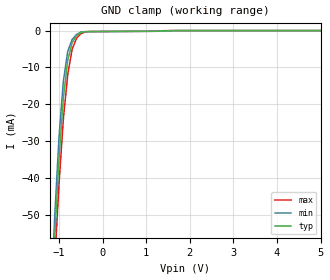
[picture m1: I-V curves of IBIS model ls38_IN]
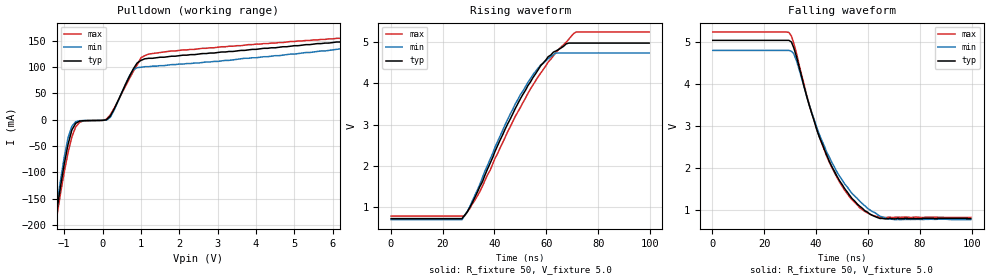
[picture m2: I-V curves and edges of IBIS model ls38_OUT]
| TEXAS INSTRUMENTS INCORPORATED
| Standard Linear and Logic Group
| IBIS Model of SN74LS38
| QUADRUPLE 2-INPUT POSITIVE-NAND BUFFERS WITH OPEN-COLLECTOR OUTPUTS
| SOP 14-pin (NS), SOIC 14-pin (D), P-DIP 14-pin (N)
[IBIS Ver]   3.2
[Comment Char] |_char
[File Name]   sn74ls38.ibs
[File Rev]   2.1 I_die
[Date]   Nov.15, 2004
[Source]   File originated at Texas Instruments, Inc.
[Notes]   The following is a sample IBIS file for the LS38.
   - FILE REV HISTORY
   - 3.2 Re-Release IBIS file on 11/16/04
   - Power clamp data deleted as there is no power-clamp diode.
|   - All test data contained in this file are derived from
|   actual measurements.
|   - File created by Nobuhisa Ohtsubo, SLL Product Engineering.
[Disclaimer] Property of Texas Instruments Incorporated.  Unauthorized
   reproduction and/or distribution is strictly prohibited.
   This product is protected under copyright law.
   Created 2000, (C) Copyright 2000, Texas Instruments Inc.,
   All Rights Reserved.
   UNLESS THERE IS A SIGNED, WRITTEN AGREEMENT TO THE
   CONTRARY, TEXAS INSTRUMENTS () IS PROVIDING THE IBIS
   MODELS  AND WITHOUT ANY WARRANTY, EXPRESSED OR
   IMPLIED.  TI assumes no liability for:
   1) the accuracy of the IBIS models provided to your
   company;
   2) the proper functioning of these IBIS Models in your
   design or for any resulting applications; or
   3) infringement of patents, copyrights or intellectual
   property rights resulting from your use of these IBIS
   models.
   TI provides IBIS Models as a service to our customers.
   You and your company shall not distribute, sell or give
   these models to anyone else without prior written
   permission from TI.
   TI reserves the right to make changes to our products or
   to discontinue any semiconductor product or service
   without notice, and advises our customers to obtain the
   latest version of relevant information to verify, before
   placing orders, that the information being relied on is
   current.
   Please be aware that your receipt and use of the IBIS
   information provided shall serve as acceptance of these
   terms and conditions.  If you do not accept these terms,
   you should return or destroy the IBIS models and any
   other accompanying information immediately.
|   Component LS38_NS
[Component]   ls38_NS
[Manufacturer]  Texas Instruments, Inc.
[Package]
|   typ   min   max
R_pkg   0.045   0.039   0.054
L_pkg   3.796nH   2.561nH   4.952nH
C_pkg   0.528pF   0.288pF   0.710pF
[Pin]   signal_name   model_name   R_pin   L_pin   C_pin
1   1A   ls38_IN   0.047   4.867nH   0.706pF
2   1B   ls38_IN   0.051   4.083nH   0.592pF
3   1Y   ls38_OUT   0.041   2.915nH   0.376pF
4   2A   ls38_IN   0.039   2.561nH   0.288pF
5   2B   ls38_IN   0.041   3.101nH   0.430pF
6   2Y   ls38_OUT   0.047   4.047nH   0.589pF
7   GND   GND   0.051   4.909nH   0.700pF
8   3Y   ls38_OUT   0.045   4.784nH   0.694pF
9   3A   ls38_IN   0.054   4.176nH   0.597pF
10   3B   ls38_IN   0.039   3.287nH   0.449pF
11   4Y   ls38_OUT   0.039   2.586nH   0.294pF
12   4A   ls38_IN   0.040   2.802nH   0.371pF
13   4B   ls38_IN   0.049   4.080nH   0.593pF
14   VCC   POWER   0.052   4.952nH   0.710pF
|   Component LS38_D
[Component]   ls38_D
[Manufacturer]  Texas Instruments, Inc.
[Package]
|   typ   min   max
R_pkg   0.031   0.028   0.034
L_pkg   3.109nH   2.462nH   3.889nH
C_pkg   0.473pF   0.363pF   0.628pF
[Pin]   signal_name   model_name   R_pin   L_pin   C_pin
1   1A   ls38_IN   0.033   3.854nH   0.622pF
2   1B   ls38_IN   0.032   3.188nH   0.473pF
3   1Y   ls38_OUT   0.028   2.462nH   0.377pF
4   2A   ls38_IN   0.031   2.596nH   0.363pF
5   2B   ls38_IN   0.028   2.521nH   0.372pF
6   2Y   ls38_OUT   0.034   3.250nH   0.476pF
7   GND   GND   0.034   3.889nH   0.628pF
8   3Y   ls38_OUT   0.034   3.889nH   0.628pF
9   3A   ls38_IN   0.034   3.250nH   0.476pF
10   3B   ls38_IN   0.028   2.521nH   0.372pF
11   4Y   ls38_OUT   0.031   2.596nH   0.364pF
12   4A   ls38_IN   0.028   2.462nH   0.377pF
13   4B   ls38_IN   0.032   3.188nH   0.473pF
14   VCC   POWER   0.033   3.854nH   0.622pF
|   Component LS38_N
[Component]   ls38_N
[Manufacturer]   Texas Instruments, Inc.
[Package]
|   typ   min   max
R_pkg   4.500e-02   3.700e-02   6.300e-02
L_pkg   5.407e-09   3.922e-09   6.942e-09
C_pkg   3.890e-13   2.050e-13   6.040e-13
[Pin]   signal_name   model_name   R_pin   L_pin   C_pin
1   1A   ls38_IN   6.300e-02   6.942e-09   6.040e-13
2   1B   ls38_IN   3.700e-02   6.200e-09   4.060e-13
3   1Y   ls38_OUT   4.200e-02   4.389e-09   3.220e-13
4   2A   ls38_IN   3.800e-02   3.922e-09   2.050e-13
5   2B   ls38_IN   3.900e-02   4.301e-09   2.980e-13
6   2Y   ls38_OUT   3.800e-02   5.329e-09   3.560e-13
7   GND   GND   5.300e-02   6.510e-09   5.440e-13
8   3Y   ls38_OUT   5.300e-02   6.437e-09   5.390e-13
9   3A   ls38_IN   3.900e-02   5.352e-09   3.470e-13
10   3B   ls38_IN   4.200e-02   4.473e-09   2.970e-13
11   4Y   ls38_OUT   4.400e-02   4.326e-09   2.250e-13
12   4A   ls38_IN   4.200e-02   4.295e-09   2.800e-13
13   4B   ls38_IN   4.200e-02   6.318e-09   4.180e-13
14   VCC   POWER   6.100e-02   6.900e-09   6.030e-13
| Models and submodels in the file (2): ls38_IN (Input), ls38_OUT (Open_drain)
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|   Model ls38_IN
[Model]   ls38_IN
Model_type  Input
Polarity   Inverting
Vinl = 0.8
Vinh = 2.0
| variable   typ   min   max
C_comp   1.33pf   1.00pf   1.66pf
[Temperature Range]   25   0   70
[Voltage Range]   5.00   4.75   5.25
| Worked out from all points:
|   GND clamp passes 1 mA (typ) near -0.55 V on its own axis
[GND Clamp]
|   Voltage   I(typ)   I(min)   I(max)
-5V       -1.27A     -1.34A     -1.18A
-1.2V     -82.8mA    -77.4mA    -88.2mA
-1.1V     -57mA      -50.9mA    -63.5mA
-1V       -34.9mA    -29mA      -41.8mA
-900mV    -18.2mA    -13.7mA    -24.1mA
-800mV    -8.05mA    -5.64mA    -12mA
-700mV    -3.3mA     -2.45mA    -5.17mA
-600mV    -1.43mA    -1.07mA    -2.13mA
-500mV    -556uA     -392uA     -875uA
-400mV    -294uA     -293uA     -355uA
-300mV    -272uA     -285uA     -257uA
5V        3.28nA     893pA      12.5nA
|   Model ls38_OUT
[Model]   ls38_OUT
Model_type  Open_drain
Polarity   Non-Inverting
Vmeas = 1.5v
Cref = 0pf
| variable   typ   min   max
C_comp   5.8pf   4.35pf   7.25pf
[Temperature Range]   25   0   70
[Voltage Range]   5.0   4.75   5.25
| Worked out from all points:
|   slope of the pulldown table from 0 to 0.75 V, typ, clamps not added: 8.26 ohm
|   rising waveform, R_fixture 50, V_fixture 5.0: 20-80 % time 19.7ns typ, 18ns min, 22.4ns max; typ from 0.722 V to 4.98 V
|   falling waveform, R_fixture 50, V_fixture 5.0: 20-80 % time 15.3ns typ, 16.5ns min, 14.8ns max; typ from 5.04 V to 0.782 V
[Pulldown]
|   Voltage   I(typ)   I(min)   I(max)
-5V       -2.01A     -2.11A     -1.91A
-1.3V     -226mA     -219mA     -233mA
-1.2V     -177mA     -168mA     -188mA
-1V       -84.8mA    -71.5mA    -100mA
-800mV    -19.5mA    -12.5mA    -32.6mA
-600mV    -2.64mA    -1.88mA    -4.95mA
100mV     -170uA     -759uA     989uA
300mV     20.1mA     18mA       21.6mA
800mV     96.6mA     95.1mA     91.8mA
1V        113mA      100mA      118mA
1.2V      117mA      101mA      125mA
10V       177mA      172mA      176mA
[Ramp]
| variable   typ   min   max
dV/dt_r   2.502/19.13n   2.364/17.27n   2.658/21.86n
dV/dt_f   2.616/15.62n   2.478/19.91n   2.718/15.14n
R_load = 50
[Rising Waveform]
R_fixture = 50
V_fixture = 5.0
V_fixture_min = 4.75
V_fixture_max = 5.25
C_fixture = 0pf
L_fixture = 0nH
|   Time   V(typ)   V(min)   V(max)
195ps     722mV      696mV      783mV
27.5ns    722mV      696mV      783mV
28.5ns    803mV      796mV      785mV
34.4ns    1.5V       1.56V      1.38V
44.1ns    2.89V      3V         2.69V
50ns      3.63V      3.73V      3.42V
57.8ns    4.43V      4.45V      4.25V
62.7ns    4.76V      4.7V       4.67V
71.5ns    4.98V      4.74V      5.25V
99.6ns    4.98V      4.74V      5.25V
[Falling Waveform]
R_fixture = 50
V_fixture = 5.0
V_fixture_min = 4.75
V_fixture_max = 5.25
|   Time   V(typ)   V(min)   V(max)
195ps     5.04V      4.8V       5.24V
29.5ns    5.04V      4.8V       5.23V
30.5ns    5V         4.78V      5.14V
32.4ns    4.66V      4.56V      4.74V
37.3ns    3.5V       3.51V      3.52V
44.1ns    2.3V       2.37V      2.27V
51ns      1.5V       1.61V      1.46V
56.8ns    1.08V      1.2V       1.04V
67.6ns    781mV      777mV      815mV
99.6ns    782mV      761mV      813mV
